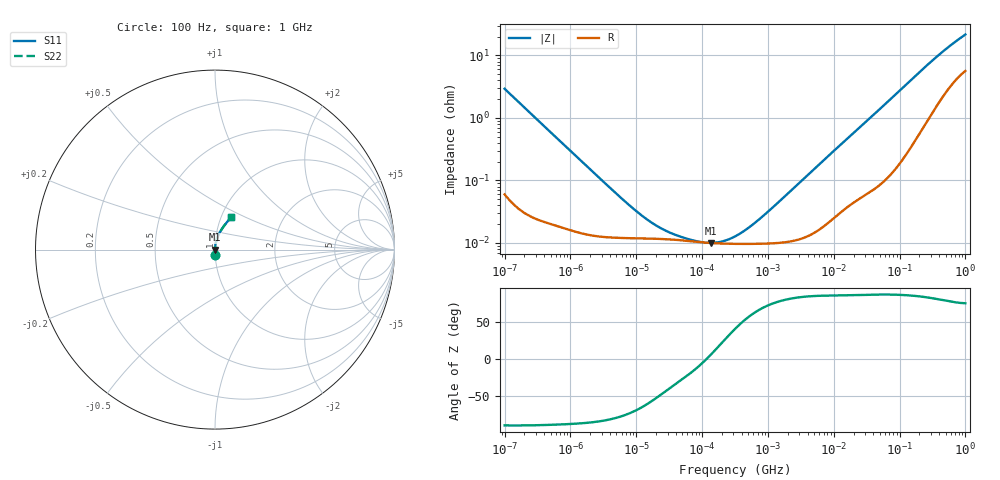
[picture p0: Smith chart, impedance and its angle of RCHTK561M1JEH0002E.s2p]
! RCHTK561M1JEH0002E  S-PARAMETER MODEL  (AEC-Q200 qualified)
! Model Generated by ELNA Corporation (http://www.ty-top.com)
! Version 1.0
! ELNA Control No.240315
! Copyright (c) 2024 ELNA CO.,LTD. All Rights Reserved.
! Products Name : CONDUCTIVE POLYMER HYBRID ALUMINUM ELECTROLYTIC CAPACITORS
! Characteristics :
!  Capacitance  :  560uF  ,  Rated voltage  :  6.3V
!  Operating Temp. Range  :  -55 to +125 degC  ,  Endurance  :  4000hr at 125 degC
!  Dimension D  :  8mm  ,  Dimension L  :  10mm
! Frequency Range : 100Hz - 1GHz
! External Node Assignments :
!  1  o---| |---o  2
# MHz S RI R 50
!Freq[MHz].  S11 Real  S11 Imag  S21 Real  S21 Imag  S12 Real  S12 Imag  S22 Real  S22 Imag
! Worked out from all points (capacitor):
!   401 points, 100 Hz to 1 GHz, reference 50 ohm
!   read as one part in series: C = 543 uF near 108 Hz
!   lowest |Z| = 10 mohm at 135.7 kHz (marker M1)
!   series resonance near 116.5 kHz, so ESL is about 3.4 nH
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0.0001  0.00145 -0.0292  0.9985 0.0292  0.9985 0.0292  0.00145 -0.0292
0.000113  0.00119 -0.0259  0.9988 0.0259  0.9988 0.0259  0.00119 -0.0259
0.001488  0.000146 -0.00201  0.9999 0.00201  0.9999 0.00201  0.000146 -0.00201
0.004597  0.000122 -0.000653  0.9999 0.000653  0.9999 0.000653  0.000122 -0.000653
0.008414  0.000119 -0.000357  0.9999 0.000357  0.9999 0.000357  0.000119 -0.000357
0.014207  0.000118 -0.000212  0.9999 0.000212  0.9999 0.000212  0.000118 -0.000212
0.022131  0.000116 -0.000136  0.9999 0.000136  0.9999 0.000136  0.000116 -0.000136
0.034475  0.000113 -8.62e-05  0.9999 8.62e-05  0.9999 8.62e-05  0.000113 -8.62e-05
0.055911  0.000109 -4.8e-05  0.9999 4.8e-05  0.9999 4.8e-05  0.000109 -4.8e-05
0.090678  0.000103 -1.63e-05  0.9999 1.63e-05  0.9999 1.63e-05  0.000103 -1.63e-05
0.135675  9.99e-05 1.03e-05  0.9999 -1.03e-05  0.9999 -1.03e-05  9.99e-05 1.03e-05
0.203002  9.78e-05 4.05e-05  0.9999 -4.05e-05  0.9999 -4.05e-05  9.78e-05 4.05e-05
0.316228  9.67e-05 8.24e-05  0.9999 -8.24e-05  0.9999 -8.24e-05  9.67e-05 8.24e-05
0.473151  9.65e-05 0.000135  0.9999 -0.000135  0.9999 -0.000135  9.65e-05 0.000135
0.767361  9.71e-05 0.000228  0.9999 -0.000228  0.9999 -0.000228  9.71e-05 0.000228
1.40443  0.0001 0.000424  0.9999 -0.000424  0.9999 -0.000424  0.0001 0.000424
4.704354  0.000141 0.00142  0.9999 -0.00142  0.9999 -0.00142  0.000141 0.00142
69.9842  0.00155 0.0192  0.9985 -0.0192  0.9985 -0.0192  0.00155 0.0192
169.8244  0.00628 0.0454  0.9937 -0.0454  0.9937 -0.0454  0.00628 0.0454
365.1741  0.0236 0.0903  0.9764 -0.0903  0.9764 -0.0903  0.0236 0.0903
641.9482  0.0541 0.1371  0.9459 -0.1371  0.9459 -0.1371  0.0541 0.1371
1000  0.0893 0.1802  0.9107 -0.1802  0.9107 -0.1802  0.0893 0.1802
